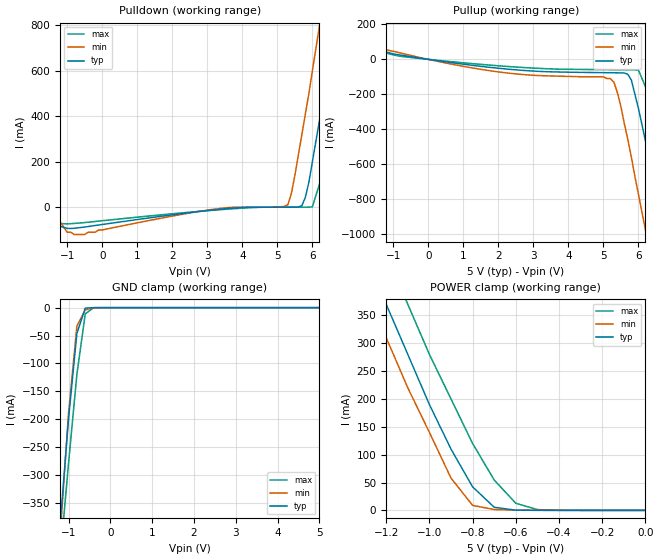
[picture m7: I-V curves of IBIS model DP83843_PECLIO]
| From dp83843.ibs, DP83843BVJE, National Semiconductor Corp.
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|   Model PECLIO
[Model]   DP83843_PECLIO
Model_type   I/O
Polarity   Non-Inverting
Enable   Active-High
Vinl =   0.50V
Vinh =   4.50V
Vmeas =   2.50V
Cref =  10.00pF
Rref =  50.00
C_comp   5.00pF   5.00pF   5.00pF
[Temperature Range]   50.00   -15.00   0.15k
[Voltage Range]   5.00V   4.50V   5.50V
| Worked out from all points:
|   slope of the pulldown table from 0 to 0.75 V, typ, clamps not added: 45.8 ohm
|   slope of the pullup table from 0 to 0.75 V, typ, clamps not added: 35.6 ohm
|   GND clamp passes 1 mA (typ) near -0.60 V on its own axis
|   POWER clamp passes 1 mA (typ) near -0.61 V on its own axis
[Pulldown]
| voltage   I(typ)   I(min)   I(max)
-5V       -19.35mA   -16.78mA   -27.02mA
-1.8V     -14.32mA   -16.26mA   -56.99mA
-1.4V     -75.9mA    -20.17mA   -70.17mA
-500mV    -87.08mA   -120mA     -67.57mA
5.2V      29.16nA    3.17mA     4.79nA
5.4V      8.37uA     60.43mA    9.52nA
5.7V      6.65mA     320mA      770nA
6V        200mA      600mA      1.82mA
6.4V      560mA      990mA      200mA
6.8V      940mA      1.39A      560mA
7.2V      1.33A      1.8A       930mA
10V       4.16A      4.67A      3.7A
[Pullup]
| voltage   I(typ)   I(min)   I(max)
-5V       160mA      150mA      170mA
-2.6V     110mA      130mA      93.35mA
-500mV    15.1mA     22.55mA    10.57mA
2.2V      -54.62mA   -76.58mA   -39.68mA
5.2V      -76.6mA    -110mA     -59.08mA
5.4V      -77.11mA   -190mA     -59.41mA
5.7V      -85.89mA   -460mA     -59.88mA
6V        -280mA     -770mA     -61.46mA
6.4V      -650mA     -1.18A     -250mA
6.8V      -1.04A     -1.59A     -600mA
7.2V      -1.43A     -2A        -970mA
10V       -4.19A     -4.78A     -3.67A
[GND_clamp]
| voltage   I(typ)   I(min)   I(max)
-5V       -4.19A     -4.3A      -4.16A
-1.2V     -390mA     -410mA     -450mA
-1V       -200mA     -190mA     -280mA
-800mV    -46.37mA   -33.01mA   -120mA
-600mV    -760uA     -4.15mA    -11.16mA
-400mV    -4.92uA    -120uA     -82.71uA
5V        1.06nA     180uA      7.23nA
[POWER_clamp]
| voltage   I(typ)   I(min)   I(max)
-5V       4.13A      4.13A      4.17A
-1.3V     460mA      410mA      550mA
-1.2V     370mA      310mA      460mA
-1.1V     280mA      220mA      370mA
-1V       190mA      140mA      280mA
-900mV    110mA      57.98mA    200mA
-800mV    42.21mA    8.93mA     120mA
-700mV    5.57mA     1.46mA     54.46mA
-600mV    330uA      390uA      12.72mA
-500mV    38.48uA    180uA      1.38mA
0V        1.06nA     1.44nA     10.48nA
[Ramp]
| variable   typ   min   max
dV/dt_r   0.55/0.31n   0.58/0.21n   0.49/0.43n
dV/dt_f   0.17m/7.50p   0.17m/6.57p   0.23m/11.98p
R_load = 50.00
| End [Model] PECLIO
